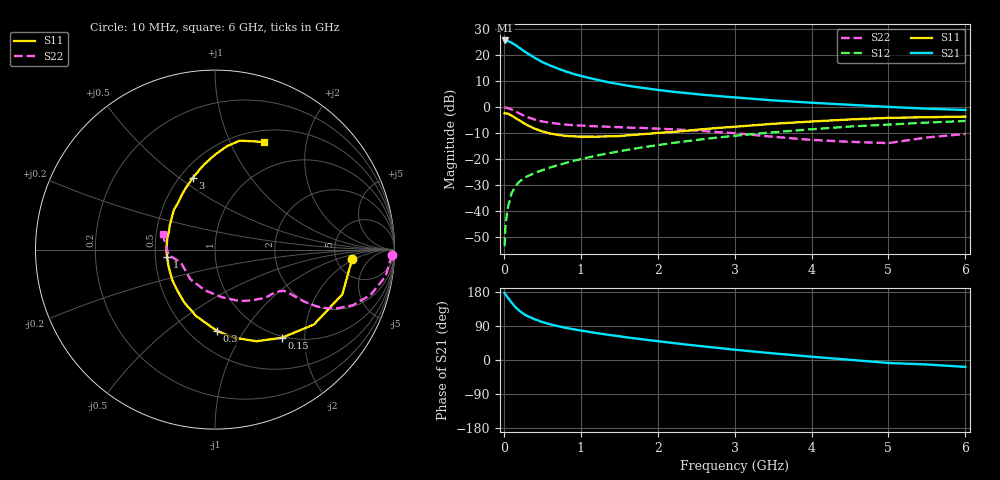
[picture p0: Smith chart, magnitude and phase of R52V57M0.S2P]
! SIEMENS Small Signal Semiconductors
! BFR183
! Si NPN RF Bipolar Junction Transistor in SOT23
! VCE = 2.5 V  IC = 7 mA
! Common Emitter S-Parameters:  May  1996
# GHz  S  MA  R  50
!  f  S11  S21  S12  S22
! GHz  MAG  ANG  MAG  ANG  MAG  ANG  MAG  ANG
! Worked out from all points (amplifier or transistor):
!   36 points, 10 MHz to 6 GHz, reference 50 ohm
!   highest |S21| = 25.7 dB at 20 MHz (marker M1)
!   |S21| within 3 dB of that: start of sweep to 209.9 MHz
!   unconditionally stable (mu >= 1): 883.6 MHz to 2.562 GHz
!   at 250 MHz: K = 0.51, MSG = 24.7 dB, |S12| = -27.6 dB
!   at 1.4 GHz: K = 1.06, MAG = 11.9 dB, |S12| = -17.6 dB
!   at 6 GHz: K = 0.89, MSG = 2.1 dB, |S12| = -5.3 dB
!   lowest NFmin = 1.25 dB at 450 MHz
!   S11 on the Smith chart (normalised r, x): 10 MHz: 7.04, -1.86; 150 MHz: 0.97, -1.54; 300 MHz: 0.67, -0.77; 1 GHz: 0.58, -0.05; 3 GHz: 0.58, +0.56; 6 GHz: 0.64, +1.35
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0.01  0.7658 -4.1  19.16 177.0  0.0021 88.6  0.986 -1.7
0.02  0.7569 -7.9  19.24 173.7  0.0049 83.5  0.9784 -3.6
0.05  0.7522 -19.3  18.84 165.1  0.0113 80.8  0.9621 -8.9
0.1  0.6917 -37.1  17.47 151.7  0.0218 73.7  0.9024 -16.3
0.15  0.6162 -52.9  15.75 139.5  0.0301 66.9  0.8278 -22.0
0.2  0.5598 -65.8  13.95 130.5  0.0364 63.4  0.7584 -25.5
0.25  0.5 -78.3  12.36 122.7  0.0418 61.2  0.6987 -27.8
0.3  0.4533 -88.6  11.04 116.5  0.0462 59.7  0.6486 -29.2
0.4  0.3852 -105.7  8.932 107.7  0.0539 59.0  0.5765 -30.2
0.5  0.3416 -119.9  7.386 100.2  0.0611 58.8  0.53 -30.4
0.6  0.3102 -132.5  6.346 94.4  0.0686 59.6  0.5007 -30.4
0.7  0.2931 -143.9  5.555 89.4  0.076 60.6  0.4782 -30.4
0.8  0.2797 -154.1  4.899 85.1  0.0837 61.0  0.4611 -30.6
1  0.2701 -171.1  3.997 77.8  0.0996 61.6  0.4419 -31.3
1.1  0.2708 -178.8  3.677 74.5  0.1078 62.0  0.4343 -32.3
1.6  0.2859 151.9  2.604 59.7  0.1498 61.0  0.4039 -37.5
2.2  0.3318 128.4  1.977 44.9  0.2047 57.5  0.3739 -47.0
3  0.4187 107.2  1.54 27.2  0.2814 49.8  0.3146 -65.2
3.5  0.4777 97.4  1.35 17.5  0.3272 43.9  0.2689 -81.5
4.5  0.5798 83.4  1.109 0.5  0.4235 31.6  0.2148 -130.3
5.5  0.6392 70.8  0.934 -11.8  0.5042 19.5  0.2606 -173.7
6  0.6577 65.7  0.882 -18.2  0.5417 11.5  0.3044 163.7
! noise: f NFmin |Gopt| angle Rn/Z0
0.45  1.25  0.18  42  0.22
0.9  1.3  0.22  110  0.2
1.8  2  0.33  180  0.14
